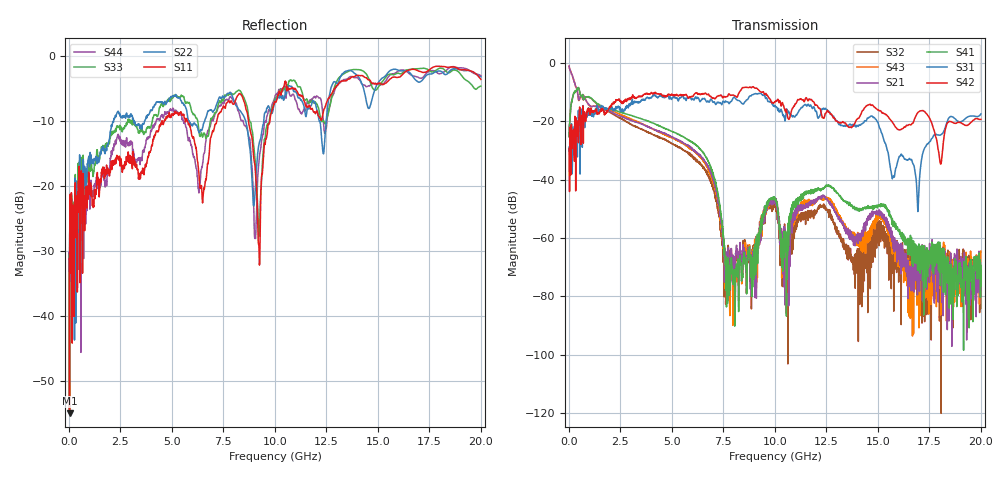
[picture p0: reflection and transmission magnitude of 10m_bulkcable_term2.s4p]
# MHz S MA R 50.00
! FREQ  S11  S12  S13  S14
!  S21  S22  S23  S24
!  S31  S32  S33  S34
!  S41  S42  S43  S44
!  MAG  ANG  MAG  ANG  MAG  ANG  MAG  ANG
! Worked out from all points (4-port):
!   2000 points, 10 MHz to 20 GHz, reference 50 ohm
!   strongest paths, dB at 10 MHz, 5.01 GHz, 10.01 GHz, 15.01 GHz, 20 GHz:
!     S42: -29.3, -10.8, -13.4, -16.1, -19.4
!     S31: -28.8, -12.1, -14.7, -20.5, -17.5
!     S41: -25.3, -23.5, -46.9, -48.8, -76.4
!     S21: -1.2, -25.5, -46.7, -51.0, -76.9
!     S43: -1.2, -25.7, -47.0, -53.7, -64.5
!     S32: -25.3, -27.6, -47.5, -58.6, -77.9
!   lowest |S11| = -55.0 dB at 30 MHz (marker M1), VSWR 1.00, Z = 49.9 + j0.148 ohm
!   |S11| at or under -10 dB: start of sweep to 4.52 GHz; 5.746 GHz to 7.176 GHz (1.431 GHz wide, 22.1 % of centre); 8.714 GHz to 9.76 GHz (1.046 GHz wide, 11.3 % of centre)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
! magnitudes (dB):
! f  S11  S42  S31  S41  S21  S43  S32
! 10 MHz  -31.3  -29.3  -28.8  -25.3  -1.2  -1.2  -25.3
! 30 MHz  -55.0  -44.1  -37.0  -21.0  -2.0  -2.0  -21.0
! 6.25 GHz  -16.3  -10.8  -11.9  -28.5  -31.1  -31.4  -33.7
! 8.05 GHz  -7.2  -11.3  -11.9  -90.2  -72.8  -80.5  -71.7
! 12.58 GHz  -6.7  -16.6  -16.8  -41.9  -47.1  -46.4  -51.1
! 16.93 GHz  -2.3  -17.2  -50.2  -71.1  -63.6  -72.4  -79.2
! 20 GHz  -3.6  -19.4  -17.5  -76.4  -76.9  -64.5  -77.9
